// 该功能块可以对EtherCAT从站进行检测，检测内容详见 EC_SLAVE_DIAG_INFO_DATA
{attribute 'no_check'}
{attribute 'enable_dynamic_creation'}
FUNCTION_BLOCK FB_EcSlavesDiag 
VAR_INPUT
	Execute													:	BOOL := FALSE; 		// 如果为TRUE，则执行功能块
	MasterAmsNetId											:	T_AmsNetId;
END_VAR
VAR_OUTPUT
	ExecutionTime											: 	TIME;
	NoOfSlaves												:	UINT;			
    InfoData												:	ARRAY [MIN_SLAVES..MAX_SLAVES] OF EC_SLAVE_DIAG_INFO_DATA; 
	
	Busy													: BOOL; 			// 如果为TRUE，则功能块忙碌
	Done													: BOOL; 			// 如果为TRUE，则功能块完成
	Error													: BOOL;				// 如果为TRUE，则功能块存在错误
{attribute 'displaymode':='hex'}  
	ErrorId													: UDINT; 			// 错误ID
END_VAR
VAR
    {attribute 'hide'} 
	State													: INT := 0;
    {attribute 'hide'} 
	rtExecute												: R_TRIG;		

	StartTime												:	TIME;	

	pMemory													:	POINTER TO BYTE;
	SizeOfMemory											:	UDINT;

	pScannedSlaves											:	POINTER TO ARRAY [MIN_SLAVES..MAX_SLAVES] OF Tc2_EtherCAT.ST_EcSlaveScannedData;
	pConfigSlaves											:	POINTER TO ARRAY [MIN_SLAVES..MAX_SLAVES] OF Tc2_EtherCAT.ST_EcSlaveConfigData; 
	pSlavesState											:	POINTER TO ARRAY [MIN_SLAVES..MAX_SLAVES] OF Tc2_EtherCAT.ST_EcSlaveState;
	pSlavesStatusCode										:	POINTER TO ARRAY [MIN_SLAVES..MAX_SLAVES] OF DWORD;
	
(* dummy **********************************************************)
	i,k,idx													:	UINT := 0;
	
(* function-blocks *************************************************)
	EcGetSlaveCount											:	FB_EcGetSlaveCount ;
	EcGetConfSlaves											:	FB_EcGetConfSlaves ;
	EcGetScannedSlaves										:	FB_EcGetScannedSlaves ;
	EcGetAllSlaveStateS										:	FB_EcGetAllSlaveStateS ;
	EcGetAllSlaveCrcErrors									:	FB_EcGetAllSlaveCrcErrors ;
	EcGetAllSlaveAbnormalStateChanges						:	FB_EcGetAllSlaveAbnormalStateChanges ;	
	EcGetSlaveTopologyInfo									: 	FB_EcGetSlaveTopologyInfo ;	
END_VAR

(* Sequence *********************************)
	rtExecute(CLK := Execute);
	

	CASE State OF
	0:
		Busy 												:= FALSE;
		IF rtExecute.Q
		THEN //Clear data if FB is disabled or started
			Busy 											:= TRUE;
			Done											:= FALSE;
			Error											:= FALSE;
			Errorid											:= 0;


		//	NoOfSlavesNIO									:= 0;	


			StartTime										:= TIME();
			ExecutionTime									:= T#0MS;
			
			EcGetSlaveCount(bExecute := FALSE,sNetId := MasterAmsNetId);
			EcGetConfSlaves(bExecute := FALSE,sNetId := MasterAmsNetId);
			EcGetSlaveTopologyInfo(bExecute := FALSE,sNetId := MasterAmsNetId);
			EcGetAllSlaveStates(bExecute := FALSE, sNetId := MasterAmsNetId);
			EcGetAllSlaveCrcErrors(bExecute := FALSE,sNetId := MasterAmsNetId);
			EcGetAllSlaveAbnormalStateChanges(bExecute := FALSE,sNetId := MasterAmsNetId);
			EcGetScannedSlaves(bExecute := FALSE,sNetId := MasterAmsNetId);
			
			State										:= 1;
			
		ELSIF NOT Execute THEN
			Done											:= FALSE;
			Error											:= FALSE;
			Errorid											:= 0;

		END_IF
		IF StartTime > T#0MS AND ExecutionTime = T#0MS
		THEN
			ExecutionTime									:= TIME() - StartTime;
		END_IF
		
	(* Read no of configured slaves *********************************************************************)
	1:
		EcGetSlaveCount(bExecute := NoOfSlaves = 0);
		IF NOT EcGetSlaveCount.bBusy
		THEN
			IF EcGetSlaveCount.bError 
			THEN
				Busy										:= FALSE;
				Error										:= TRUE;
				ErrorId										:= EcGetSlaveCount.nErrId;
				State 										:= 0;
			ELSIF EcGetSlaveCount.bExecute AND NoOfSlaves <> EcGetSlaveCount.nSlaves
			THEN
				NoOfSlaves									:= EcGetSlaveCount.nSlaves;					

				//Init Info Data 	
				MEMSET(ADR(InfoData),0,SIZEOF(InfoData));

				//k 											:= NoOfSlaves + 1;
				//Set buffer lenght according to needed memory space
				EcGetConfSlaves.cbBufLen					:= SIZEOF(Tc2_EtherCAT.ST_EcSlaveConfigData) * NoOfSlaves;
				EcGetScannedSlaves.cbBufLen					:= SIZEOF(Tc2_EtherCAT.ST_EcSlaveScannedData) * NoOfSlaves;
				EcGetAllSlaveStates.cbBufLen				:= SIZEOF(Tc2_EtherCAT.ST_EcSlaveState) * NoOfSlaves;
				EcGetAllSlaveCrcErrors.cbBufLen				:= SIZEOF(DWORD) * NoOfSlaves;						
					
				//Allocate dynamic buffer memory 
				IF Allocate(MAX(MAX(EcGetConfSlaves.cbBufLen,EcGetAllSlaveCrcErrors.cbBufLen), MAX(EcGetScannedSlaves.cbBufLen,EcGetAllSlaveStateS.cbBufLen) ))
				THEN
					//Write buffer lenght per FB	
					pConfigSlaves							:= pMemory;
					pScannedSlaves							:= pMemory;
					pSlavesState							:= pMemory;
					pSlavesStatusCode						:= pMemory;	
					
					State 									:= State + 1;			
				ELSE
					Busy									:= FALSE;
					Error									:= TRUE;
					ErrorId									:= E_AdsErr.DEVICE_NOMEMORY; //No memory
					State 									:= 0;	
				END_IF

			ELSE
				State 										:= State + 1;
			END_IF
		ELSE
			;
		END_IF		
		
			(* Read slaves "configuration" ************************************************************************************************************)
	2:
		EcGetConfSlaves(bExecute := TRUE, pArrEcConfSlaveInfo := pConfigSlaves, cbBufLen := (* See State 1 *) );
			
		IF NOT EcGetConfSlaves.bBusy
		THEN
			IF EcGetConfSlaves.bError 
			THEN
				Busy										:= FALSE;
				Error										:= TRUE;
				ErrorId										:= EcGetConfSlaves.nErrorId;
				State										:= 0;     
					
			ELSIF EcGetConfSlaves.nSlaves > MAX_SLAVES
			THEN
				Busy										:= FALSE;
				Error										:= TRUE;
				ErrorId										:= E_AdsErr.DEVICE_INVALIDSIZE  ;
				State										:= 0;  					
			ELSE
				State 										:= State + 1;
			END_IF
		END_IF	
		
	3: //Fill structure	
		k													:= MIN(EcGetConfSlaves.nSlaves, NoOfSlaves);
		FOR i := MIN_SLAVES TO k DO
			InfoData[i].Addr								:= pConfigSlaves^[i].nAddr;
			InfoData[i].ConfigType							:= pConfigSlaves^[i].sType; 
			InfoData[i].ConfigName							:= DELETE(pConfigSlaves^[i].sName, LEN(InfoData[i].ConfigType) + 3 , FIND(pConfigSlaves^[i].sName,InfoData[i].ConfigType) - 1);  	
			InfoData[i].ConfigTypeIdentity					:= F_ConvProductCodeToString(pConfigSlaves^[i].stSlaveIdentity);
			InfoData[i].ConfigIdentity						:= pConfigSlaves^[i].stSlaveIdentity;		
		END_FOR
		
		State:=20;
		
		(* Read slaves "EtherCAT State and link state" ***************************************************************************************)
	20	:
		EcGetAllSlaveStateS(bExecute := NoOfSlaves > 0, pStateBuf:=  pSlavesState, cbBufLen	:= (* See State 1 *));
					
		IF NOT EcGetAllSlaveStateS.bBusy
		THEN
			IF EcGetAllSlaveStateS.bError 
			THEN
				Busy										:= FALSE;
				Error										:= TRUE;
				ErrorId										:= EcGetAllSlaveStateS.nErrId;
				State 										:= 0;
			ELSE
				k											:= MIN(EcGetAllSlaveStateS.nSlaves, NoOfSlaves);
				FOR i := MIN_SLAVES TO k DO
					InfoData[i].LinkState					:= pSlavesState^[i].linkState;
					InfoData[i].DevState					:= pSlavesState^[i].deviceState;
					InfoData[i].DevStateText				:= F_ConvSlaveStateToString(pSlavesState^[i]);
				END_FOR	

				State 										:= State + 1;
			END_IF
		ELSE
			;
		END_IF	
		
	(* Get all slaves "CRC counter" ********************************************************************)
	21:	
		EcGetAllSlaveCrcErrors(bExecute := NoOfSlaves > 0, sNetId	:= MasterAmsNetId,  pCrcErrorBuf:= pSlavesStatusCode,  cbBufLen	:= (* See State 1 *));
		IF NOT EcGetAllSlaveCrcErrors.bBusy
		THEN
			IF EcGetAllSlaveCrcErrors.bError 
			THEN
				Busy										:= FALSE;
				Error										:= TRUE;
				ErrorId										:= EcGetAllSlaveStateS.nErrId;
				
				State 										:= 0;
			ELSE
				k											:= MIN(EcGetAllSlaveCrcErrors.nSlaves, NoOfSlaves);
				FOR i := MIN_SLAVES TO k DO
					InfoData[i].CntOfCRCErrors				:= pSlavesStatusCode^[i];				
				END_FOR				
				
				State 										:= 40;
			END_IF
		ELSE
			;
		END_IF
		
	40:
	    Busy											:= FALSE;
		Done											:= TRUE;
		State											:= 0; 



	
END_CASE

METHOD PROTECTED  allocate : BOOL
VAR_INPUT 
	MemSize													:	UDINT;
END_VAR
VAR
END_VAR
IF MemSize = 0 THEN
	Allocate												:= FALSE;	
	
ELSIF pMemory = 0 THEN
	pMemory													:= __NEW(BYTE,MemSize );
	SizeOfMemory											:= MemSize;
	Allocate												:= TRUE;	
	
ELSIF MemSize > SizeOfMemory THEN
	__DELETE(pMemory);  	
	pMemory													:= __NEW(BYTE,MemSize );
	SizeOfMemory											:= MemSize;
	Allocate												:= TRUE;
	
ELSE
	Allocate												:= FALSE;
END_IF
END_METHOD

METHOD FB_exit : BOOL
VAR_INPUT
	bInCopyCode : BOOL; // if TRUE, the exit method is called for exiting an instance that is copied afterwards (online change).
END_VAR
IF NOT bInCopyCode AND pMemory <> 0
THEN //Release memory in case the PLC stopps
	__DELETE(pMemory);
	SizeOfMemory								:= 0;
END_IF
END_METHOD

METHOD FB_init : BOOL
VAR_INPUT
	bInitRetains : BOOL; // if TRUE, the retain variables are initialized (warm start / cold start)
	bInCopyCode : BOOL;  // if TRUE, the instance afterwards gets moved into the copy code (online change)
END_VAR
MasterAmsNetId:='5.18.64.212.2.1';
END_METHOD

END_FUNCTION_BLOCK
